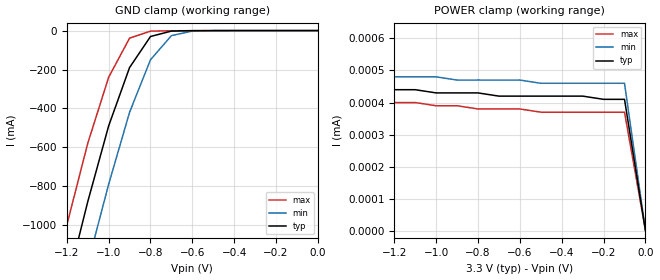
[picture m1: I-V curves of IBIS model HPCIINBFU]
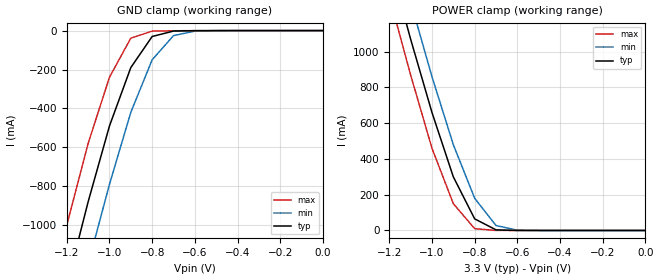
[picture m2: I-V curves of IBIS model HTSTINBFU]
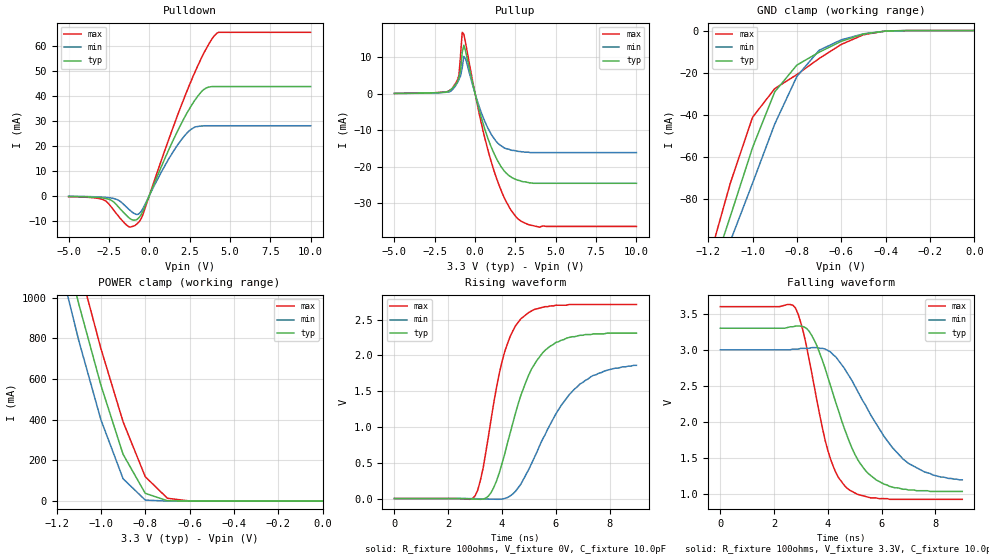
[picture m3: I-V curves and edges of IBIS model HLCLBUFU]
[IBIS Ver]   3.2
[File name]   82559erp.ibs
[File Rev]   0.0
[Date]   April 02, 2000.
[Source]   From silicon level model at Intel Corporation.
[Notes]   This file models the following:
   1. PCI   interface
   2. LOCAL/FLASH/MII   interface
   3. SMB interface
   4. LED's drivers
   It does not model the ANALOG side,
   (i.e. analog pins/balls are not part of this model).
[Disclaimer]   Data is for modeling purposes only and is not guaranteed
[Copyright]   Copyright 2000, Intel Corporation, All Rights Reserved.
[Component]   82559s
[Manufacturer] Intel Corp.
[Package]
|   typ   min   max
R_pkg   115mOhm  100mOhm  140mOhm
L_pkg   4.2nH   3.2nH   5.4nH   | rem : Mutual 1.7nH
C_pkg   0.7pF   0.4pF   1.0pF   | rem : Mutual 0.8pF
[Pin] signal_name   model_name
A1   NC   NC
A2   SERR#   HPCIODBFU
A3   VCCPP   POWER
A4   IDSEL   HPCIINBFU
A5   AD25   HPCIADBFUS
A6   PME#   HPCIODASBF
A7   VCCPP   POWER
A8   AD30   HPCIADBFUS
A9   ALTRST#   HPCIINBFU
A10   SMBCK   HSMBODBFU
A11   VCCPT   POWER
A12   LILED   YPLEDBUF
A13   TEST   HPCITSTINBFU
A14   NC   NC
B1   AD22   HPCIADBFUS
B2   AD23   HPCIADBFUS
B3   VSSPP   GND
B4   AD24   HPCIADBFUS
B5   AD26   HPCIADBFUS
B6   AD27   HPCIADBFUS
B7   VSSPP   GND
B8   AD31   HPCIADBFUS
B9   ISOLATE#   HPCIINBFU
B10   SMBALRT#   HSMBODBFU
B11   SPEEDLED   YPLEDBUF
B12   TO   HLCLBUFU
|B13  RBIAS100   ANALOG  | Not in this model.
|B14  RBIAS10   ANALOG  | Not in this model.
C1   AD21   HPCIADBFUS
C2   RST#   HPCIINBFU
C3   REQ#   HPCICMDBFU
C4   CBE#3   HPCICBEBFUS
C5   CSTSCHG   HPCIADASBF
C6   AD28   HPCIADBFUS
C7   AD29   HPCIADBFUS
C8   CLKRUN#   HPCIODABFU
C9   SMBD   HSMBODBFU
C10   VSSPT   GND
C11   ACTLED   YPLEDBUF
|C12  VREF   ANALOG  | Not in this model.
|C13  TDP   ANALOG  | Not in this model.
|C14  TDN   ANALOG  | Not in this model.
D1   AD18   HPCIADBFUS
D2   AD19   HPCIADBFUS
D3   AD20   HPCIADBFUS
D4   VSS   GND
D5   VSS   GND
D6   VSS   GND
D7   VSS   GND
D8   VSS   GND
D9   NC   NC
D10   NC   NC
D11   VSS   GND
D12   TI   HTSTINBFU
D13   TEXEC   HTSTINBFU
D14   TCK   HTSTINBFU
E1   VCCPP   POWER
E2   VSSPP   GND
E3   AD17   HPCIADBFUS
E4   VSS   GND
E5   VSS   GND
E6   VSS   GND
E7   VSS   GND
E8   VSS   GND
E9   VSS   GND
E10   VSS   GND
E11   VSS   GND
E12   VCCT   POWER
|E13  RDP   ANALOG  | Not in this model.
|E14  RDN   ANALOG  | Not in this model.
F1   IRDY#   HPCICMDBFU
F2   FRAME#   HPCICMDBFU
F3   CBE#2   HPCICBEBFUS
F4   VSS   GND
F5   VSS   GND
F6   VSS   GND
F7   VSS   GND
F8   VSS   GND
F9   VSS   GND
F10   VSS   GND
F11   VSS   GND
F12   FLD2   HLCLBUFUCF
F13   FLD1   HLCLBUFUCF
F14   FLD0   HLCLBUFUCF
G1   CLK   HPCICLKBF
|G2   VIO   POWER_REF  Special ref voltage 3.3v in CB mode.
G3   TRDY#   HPCICMDBFU
G4   NC   NC
G5   VCC   POWER
G6   VCC   POWER
G7   VSS   GND
G8   VSS   GND
G9   VSS   GND
G10   VSS   GND
G11   VSS   GND
G12   FLD3   HLCLBUFUCF
G13   VCCPL   POWER
G14   VSSPL   GND
H1   STOP#   HPCICMDBFU
H2   INTA#   HPCIODBFU
H3   DEVSEL#   HPCICMDBFU
H4   NC   NC
H5   VCC   POWER
H6   VCC   POWER
H7   VCC   POWER
H8   VCC   POWER
H9   VSS   GND
H10   VSS   GND
H11   VSS   GND
H12   FLD6   HLCLBUFUCF
H13   FLD5   HLCLBUFUCF
H14   FLD4   HLCLBUFUCF
J1   PAR   HPCICMDBFU
J2   PERR#   HPCICMDBFU
J3   GNT#   HPCIINBFU
J4   NC   NC
J5   VCC   POWER
J6   VCC   POWER
J7   VCC   POWER
J8   VCC   POWER
J9   VCC   POWER
J10   VCC   POWER
J11   VCC   POWER
J12   FLA1   HLCLBUFUCF
J13   FLA0   HLCLBUFUCF
J14   FLD7   HLCLBUFUCF
K1   AD16   HPCIADBFUS
K2   VSSPP   GND
K3   VCCPP   POWER
K4   VCC   POWER
K5   VCC   POWER
K6   VCC   POWER
K7   VCC   POWER
K8   VCC   POWER
K9   VCC   POWER
K10   VCC   POWER
K11   VCC   POWER
K12   VSSPL   GND
K13   VCCPL   POWER
K14   FLA2   HLCLBUFUCF
L1   AD14   HPCIADBFUS
L2   AD15   HPCIADBFUS
L3   CBE#1   HPCICBEBFUS
L4   VCC   POWER
L5   VCC   POWER
L6   VSS   GND
L7   CFCS#   HLCLBUFUCFIBEN
L8   CFCLK   HLCLBUFUCLKCF
L9   VCC   POWER
L10   VCC   POWER
L11   VSS   GND
L12   FLA5   HLCLBUFU
L13   FLA4   HLCLBUFU
L14   FLA3   HLCLBUFUCF
M1   AD11   HPCIADBFUS
M2   AD12   HPCIADBFUS
M3   AD13   HPCIADBFUS
M4   CBE#0   HPCICBEBFUS
M5   AD5   HPCIADBFUS
M6   VSSPP   GND
M7   AD1   HPCIADBFUS
M8   FLOE#   HLCLBUFUCF
M9   FLWE#   HLCLBUFUPCF
M10   FLA15/EESK   HLCLBUFUCF
M11   FLA12   HLCLBUFU
M12   FLA11   HLCLBUFUPCF
M13   FLA7   HLCLBUFUCF
M14   FLA6   HLCLBUFU
N1   VSSPP   GND
N2   AD10   HPCIADBFUS
N3   AD9   HPCIADBFUS
N4   AD7   HPCIADBFUS
N5   AD4   HPCIADBFUS
N6   VCCPP   POWER
N7   AD0   HPCIADBFUS
N8   VCCPL   POWER
N9   FLCS#   HLCLBUFU
N10   FLA14/EEDO   HLCLBUFUCF
|N11  X1   ANALOG   | Not in this model.
N12   VSSPL   GND
N13   FLA10   HLCLBUFUCF
N14   FLA8/IOCHRDY  HLCLBUFUCF
P1   NC   NC
P2   VCCPP   POWER
P3   AD8   HPCIADBFUS
P4   AD6   HPCIADBFUS
P5   AD3   HPCIADBFUS
P6   AD2   HPCIADBFUS
P7   EECS   HLCLBUFU
P8   VSSPL   GND
P9   FLA16   HLCLBUFU
P10   FLA13/EEDI   HLCLBUFUCF
|P11  X2   ANALOG   | Not in this model.
P12   VCCPL   POWER
P13   FLA9   HLCLBUFUCF
P14   NC   NC
| Models and submodels in the file (18): HPCIINBFU (Input), HPCICLKBF (Input), HPCITSTINBFU (Input), HTSTINBFU (Input), HLCLBUFU (I/O), HLCLBUFUCF (I/O), HLCLBUFUPCF (I/O), HLCLBUFUCFIBEN (I/O), HLCLBUFUCLKCF (I/O), HPCIADBFUS (I/O), HPCICBEBFUS (I/O), HPCIADASBF (I/O), HPCICMDBFU (I/O), HPCIODBFU (I/O_open_drain), HPCIODABFU (I/O_open_drain), YPLEDBUF (I/O), HPCIODASBF (I/O_open_drain), HSMBODBFU (I/O_open_drain)
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[Model]   HPCIINBFU
Model_type   Input
Vinl  =   1.08V   | note : 0.3 * VCCmax
Vinh  =   1.5V   | note : 0.5 * VCCmin
|variable   typ   min   max
C_comp   2.3pF   NA   NA
| note : on die power/gnd supply distribution R/L/C
|   are not included in the simulation
| note : 0.01 OHM serial resistor added to the PAD.
| note : pull up  pmos is not active  pup#="1"
| note : POWER_clamp ref = VIO = VREF = 5V
|variable   typ   min   max
[Voltage range]   3.3V   3.0V   3.6V
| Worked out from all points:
|   GND clamp passes 1 mA (typ) near -0.62 V on its own axis
|   POWER clamp passes 1 mA (typ) near -2.33 V on its own axis
| note : all DC curves are with 0.2 OHM res. in series to the PAD.
[GND_clamp]
|Voltage   I(typ)   I(min)   I(max)
-5V       -19.8A     -20.1A     -19.6A
-1.3V     -1.76A     -2.08A     -1.44A
-1.2V     -1.31A     -1.63A     -1A
-1.1V     -880mA     -1.2A      -580mA
-1V       -490mA     -790mA     -240mA
-900mV    -190mA     -420mA     -38.8mA
-800mV    -30.4mA    -150mA     -2.82mA
-700mV    -2.53mA    -25.9mA    -960uA
-600mV    -520uA     -2.57mA    -530uA
0V        -380pA     -520pA     -550pA
[POWER_clamp]
|Voltage  I(typ)   I(min)   I(max)
-5V       11.7A      10.4A      13A
-2.3V     100uA      720nA      150mA
-2.2V     3.37uA     560nA      10.1mA
-2.1V     590nA      550nA      170uA
-2V       510nA      540nA      2.93uA
-1.9V     490nA      530nA      490nA
-1.8V     480nA      520nA      450nA
-1.4V     450nA      490nA      410nA
-800mV    430nA      470nA      380nA
-700mV    420nA      470nA      380nA
-100mV    410nA      460nA      370nA
0V        1.77nA     2.84nA     2.76nA
[Model]   HTSTINBFU
Model_type   Input
Vinl  =   1.08V   | note : 0.3 * VCCmax
Vinh  =   1.5V   | note : 0.5 * VCCmin
|variable   typ   min   max
C_comp   2.3pF   NA   NA
| note : on die power/gnd supply distribution R/L/C
|   are not included in the simulation
| note : 0.1 OHM serial resistor added to the PAD.
| note : pull up  and pull down mos are not active
|   pup#="1" pdn="0"
| note : POWER_clamp ref = VIO = VREF
|   VREF= 3.0V min.   to   3.6V max.
|variable   typ   min   max
[Voltage range]   3.3V   3.0V   3.6V
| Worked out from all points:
|   GND clamp passes 1 mA (typ) near -0.62 V on its own axis
|   POWER clamp passes 1 mA (typ) near -0.63 V on its own axis
| note : all DC curves are with 0.2 OHM res. in series to the PAD.
[GND_clamp]
|Voltage  I(typ)   I(min)   I(max)
-5V       -19.8A     -20.1A     -19.6A
-1.3V     -1.76A     -2.08A     -1.44A
-1.2V     -1.31A     -1.63A     -1A
-1.1V     -880mA     -1.2A      -580mA
-1V       -490mA     -790mA     -240mA
-900mV    -190mA     -420mA     -38.8mA
-800mV    -30.4mA    -150mA     -2.83mA
-700mV    -2.53mA    -25.9mA    -970uA
-600mV    -520uA     -2.57mA    -530uA
0V        -380pA     -520pA     -550pA
[POWER_clamp]
|Voltage  I(typ)   I(min)   I(max)
-5V       20.1A      20.3A      20A
-1.2V     1.51A      1.72A      1.31A
-1.1V     1.07A      1.28A      870mA
-1V       660mA      860mA      460mA
-900mV    300mA      480mA      150mA
-800mV    64.9mA     180mA      10.1mA
-700mV    3.5mA      27.7mA     170uA
-600mV    100uA      1.61mA     2.94uA
0V        1.77nA     2.86nA     2.76nA
[Model]   HLCLBUFU
Model_type   I/O
Vinl  =   0.8V   | note : D101S spec
Vinh  =   2V   | note : D101S spec
|variable   typ   min   max
C_comp   3.1pF   NA   NA
| note : on die power/gnd supply distribution R/L/C
|   are not included in the simulation
| note : pull up  and pull down mos are not active
|   pup#="1" pdn="0"
| note : POWER_clamp ref = VIO = VREF
|   VREF= 3.0V min.   to   3.6V max.   (connected to VCC)
|variable   typ   min   max
[Voltage range]   3.3V   3.0V   3.6V
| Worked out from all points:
|   slope of the pulldown table from 0 to 0.495 V, typ, clamps not added: 63.8 ohm
|   slope of the pullup table from 0 to 0.495 V, typ, clamps not added: 60.6 ohm
|   GND clamp passes 1 mA (typ) near -0.45 V on its own axis
|   POWER clamp passes 1 mA (typ) near -0.66 V on its own axis
|   rising waveform, R_fixture 100ohms, V_fixture 0V, C_fixture 10.0pF: 20-80 % time 1.18ns typ, 1.65ns min, 857ps max; typ from 0 V to 2.31 V
|   falling waveform, R_fixture 100ohms, V_fixture 3.3V, C_fixture 10.0pF: 20-80 % time 1.29ns typ, 1.83ns min, 926ps max; typ from 3.3 V to 1.03 V
| note : all DC curves are with 0.2 OHM res. in series to the PAD.
[GND_clamp]
|Voltage   I(typ)   I(min)   I(max)
-5V       -1.63A     -1.47A     -1.85A
-1.2V     -120mA     -130mA     -110mA
-1.1V     -88.2mA    -100mA     -72.4mA
-1V       -55.6mA    -72.5mA    -41.2mA
-900mV    -29.1mA    -44.4mA    -27.6mA
-800mV    -16.4mA    -21.8mA    -20.9mA
-700mV    -10.3mA    -9.39mA    -13.3mA
-600mV    -5.12mA    -4.42mA    -6.6mA
-500mV    -1.67mA    -1.57mA    -2mA
-400mV    -240uA     -300uA     -220uA
0V        0A         0A         0A
[PullDown]
|Voltage  I(typ)   I(min)   I(max)
-5V       -320uA     -230uA     -400uA
-2.8V     -1.01mA    -630uA     -1.76mA
-2.2V     -2.55mA    -1.14mA    -5.85mA
-1.4V     -8.01mA    -4.64mA    -11.8mA
-900mV    -9.77mA    -7.25mA    -12mA
-400mV    -6.32mA    -5.21mA    -7.64mA
1.2V      18.3mA     14.7mA     22.4mA
2.2V      31.5mA     24.1mA     39.7mA
3.3V      42.1mA     27.9mA     56mA
4V        43.7mA     28mA       63.8mA
4.3V      43.7mA     28mA       65.4mA
10V       43.7mA     28mA       65.4mA
[POWER_clamp]
|Voltage  I(typ)   I(min)   I(max)
-5V       20A        19.9A      20.2A
-1.2V     1.41A      1.23A      1.6A
-1.1V     970mA      790mA      1.16A
-1V       570mA      400mA      750mA
-900mV    230mA      110mA      390mA
-800mV    38.5mA     5.23mA     120mA
-700mV    1.75mA     120uA      14mA
-600mV    72.2uA     5.85uA     820uA
0V        1.93uA     1.69uA     2.17uA
[PullUp]
|Voltage  I(typ)   I(min)   I(max)
-5V       97.3uA     74.4uA     100uA
-1.4V     1.53mA     1.16mA     1.52mA
-1V       4.52mA     3.93mA     5.14mA
-800mV    11.3mA     7.1mA      16.8mA
-700mV    13.3mA     10.2mA     16.3mA
-600mV    11.8mA     9.65mA     14.1mA
300mV     -5.18mA    -4.13mA    -6.38mA
1.1V      -15.6mA    -11.8mA    -20.1mA
1.8V      -21.1mA    -14.8mA    -28.4mA
2.6V      -23.6mA    -15.7mA    -34mA
4V        -24.5mA    -16.1mA    -36.5mA
10V       -24.5mA    -16.1mA    -36.3mA
[Ramp]
|Variable   typ   min   max
dV/dt_r   0.46/1.85n   0.38/1.51n   0.54/2.17n
dV/dt_f   1.48/2.84n   1.53/2.63n   1.46/3.06n
R_load  = 100ohms
[Rising Waveform]
|   note : pad parasitics are not incloded
R_fixture   = 100ohms
V_fixture   = 0V
C_fixture   = 10.0pF
|Time   typ(V)   min(V)   max(V)
0s        10.17nV    18.36nV    12.5nV
3ns       -7.64mV    -2.24mV    38.32mV
3.3ns     -8.1mV     -4.97mV    430mV
3.7ns     160mV      -9.56mV    1.35V
4.1ns     620mV      300uV      2.05V
4.7ns     1.44V      200mV      2.51V
5.5ns     2.03V      820mV      2.67V
6.7ns     2.26V      1.53V      2.71V
7.8ns     2.3V       1.78V      2.71V
9ns       2.31V      1.86V      2.71V
[Falling Waveform]
|   note : pad parasitics are not incloded
R_fixture   = 100ohms
V_fixture   = 3.3V
V_fixture_min   = 3.0V
V_fixture_max   = 3.6V
C_fixture   = 10.0pF
|Time   typ   min   max
0s        3.3V       3V         3.6V
2.8ns     3.33V      3.01V      3.58V
3.1ns     3.32V      3.02V      3.23V
3.3ns     3.26V      3.02V      2.87V
4ns       2.62V      2.99V      1.6V
4.4ns     2.15V      2.85V      1.22V
4.8ns     1.72V      2.63V      1.05V
5.5ns     1.28V      2.16V      950mV
6.8ns     1.06V      1.48V      920mV
9ns       1.03V      1.19V      920mV
